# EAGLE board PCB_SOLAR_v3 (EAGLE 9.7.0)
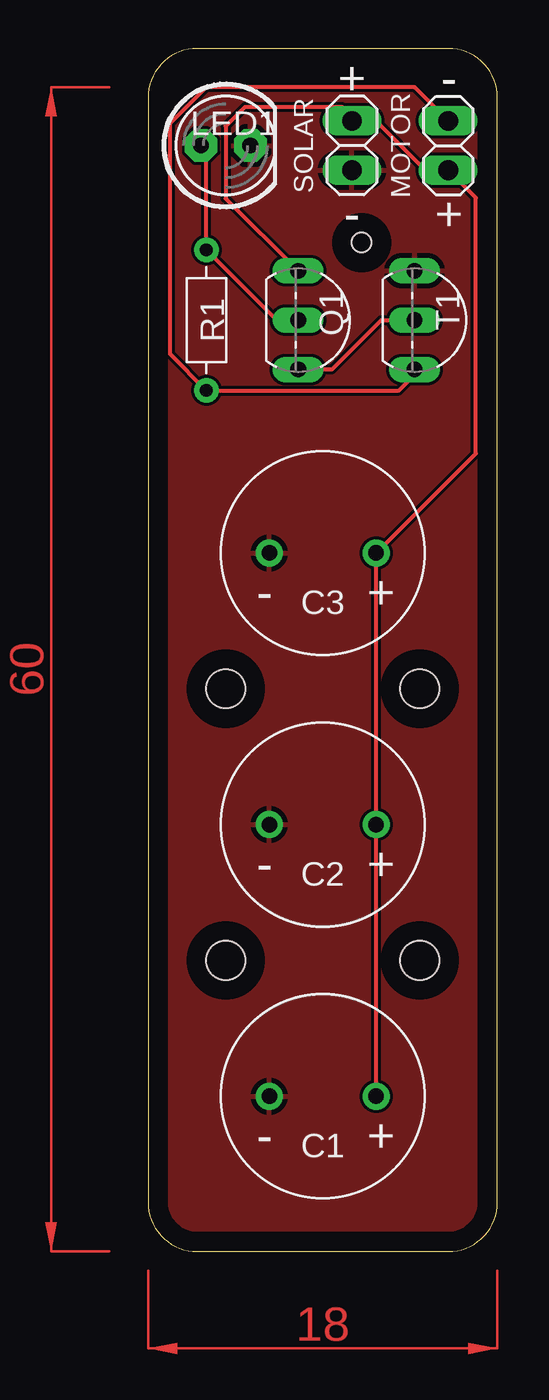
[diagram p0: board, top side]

Size 18 x 62 mm. Coordinates in mm from the lower left corner, seen from the top.
Outline: 0,59.46 0,2.54 arc90 2.54,0 15.46,0 arc90 18,2.54 18,59.46 arc90 15.46,62 2.54,62 arc90 0,59.46
Copper layers (1*16): Top 0.035mm / dielectric 1.5mm / Bottom 0.035mm
Design rules "Fusion Electronics Design Rules": minimum track width 6mil, minimum drill 0.35mm, track to track 6mil, track to pad 6mil, pad to pad 6mil, via to via 6mil, smd to smd 6mil, copper to edge 40mil, drill to drill 6mil, minimum pad ring 10mil, minimum via ring 8mil, stop-mask expansion 4mil, vias tented up to drill 0mil, thermal gap 10mil
Holes 2 mm at 4,29 14,29 4,15 14,15
Holes 1 mm at 11,52

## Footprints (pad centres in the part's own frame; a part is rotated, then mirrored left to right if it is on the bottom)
CAPRD550W60D1025H1250B = drill 0.8 pad 1.4: 1 -2.75,0; 2 2.75,0
LED5MM = drill 0.813 pad 1.676 octagon: A -1.27,0; K 1.27,0
1X02 = drill 1.016 long: 1 -1.27,0; 2 1.27,0
TO92-EBC-OVAL = drill 0.813 long: B 0,-1.27; C 2.54,-1.27; E -2.54,-1.27
RESAD724W46L381D178B = drill 0.66 pad 1.26: 1 -3.62,0; 2 3.62,0

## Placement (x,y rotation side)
C1  [CAPRD550W60D1025H1250B]  9,8 180 top
C2  [CAPRD550W60D1025H1250B]  9,22 180 top
C3  [CAPRD550W60D1025H1250B]  9,36 180 top
LED1  [LED5MM]  4,57 0 top
MOTOR  PINHD-1X02_1X02M  [1X02]  15.46,57 90 top
Q1  2N2907  [TO92-EBC-OVAL]  9,48 270 top
R1  [RESAD724W46L381D178B]  3,48 270 top
SOLAR  PINHD-1X02_1X02M  [1X02]  10.5,57 270 top
T1  2N2222  [TO92-EBC-OVAL]  15,48 270 top

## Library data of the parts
C1-C3 = Tutorial - Fusion 360; CATEGORY: Capacitor
LED1 Q1 T1 = Library
MOTOR SOLAR = Tinkercad
R1 = Tutorial - Fusion 360; CATEGORY: Resistor; SUB-CATEGORY: Fixed

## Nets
GND: C1.2 C2.2 C3.2 LED1.K SOLAR.2 T1.E
N$1: LED1.A Q1.B R1.1
N$2: C1.1 C2.1 C3.1 MOTOR.1 Q1.E SOLAR.1
N$3: MOTOR.2 R1.2 T1.C
N$5: Q1.C T1.B

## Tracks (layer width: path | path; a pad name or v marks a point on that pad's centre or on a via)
GND
  pour Top: 0,0 18,0 18,62 0,62
N$1
  Top 0.2: LED1.A 3,57 R1.1 6.62,48 Q1.B
N$2
  Top 0.2: Q1.E 4,54.27 4,58 5,59 10,59 10.5,58.5 SOLAR.1 11.73,58.27 14.27,55.73 MOTOR.1 16.88,54.31 16.88,41.13 C3.1 C2.1 C1.1
N$3
  Top 0.2: T1.C 14,45.46 12.92,44.38 R1.2 1.12,46.26 1.12,58.12 3,60 13.73,60 MOTOR.2
N$5
  Top 0.2: Q1.C 9.46,45.46 12,48 T1.B
(copper drawn outside any net)
  shapes: Top area x2

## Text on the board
tPlace: + | - | SOLAR | MOTOR | - | + | - | + | - | + | - | +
